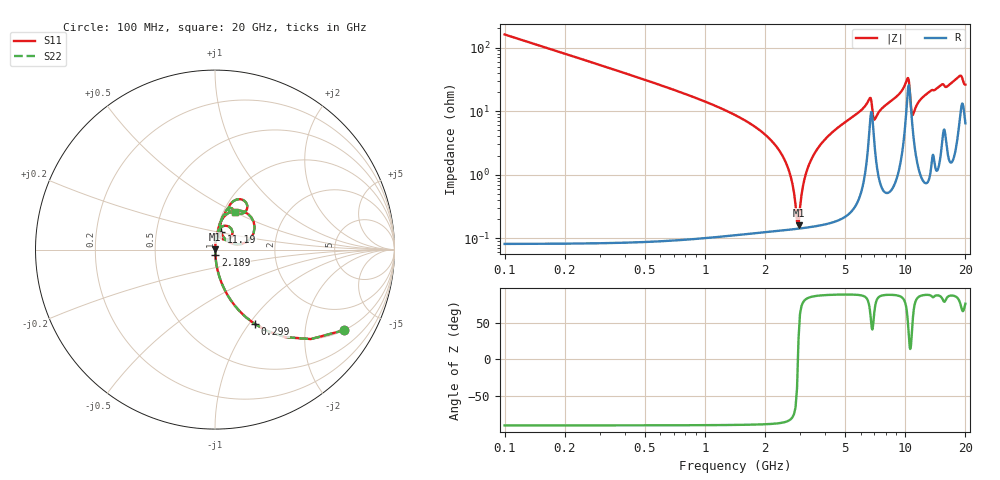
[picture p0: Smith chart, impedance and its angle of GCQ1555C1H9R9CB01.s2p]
!Murata Part Number: GCQ1555C1H9R9CB01
!These Parameters are Measured in Series Mode Connection
!Data Generated on Jan 08, 2026
!  o--ll--o
!Port1  Port2
!  o------o
!Operation Temp=25[degC], DC Bias Voltage=0[V]
!Freq. Start=100[MHz] Stop=20[GHz] 401[Steps]
# Hz S RI R 50
!Freq.(Hz) S11(Real) S11(Imag) S21(Real) S21(Imag) S12(Real) S12(Imag) S22(Real) S22(Imag)
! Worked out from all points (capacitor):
!   401 points, 100 MHz to 20 GHz, reference 50 ohm
!   read as one part in series: C = 9.9 pF near 199.5 MHz
!   lowest |Z| = 161 mohm at 2.936 GHz (marker M1)
!   series resonance near 2.916 GHz, so ESL is about 300 pH
!   S11 on the Smith chart (normalised r, x): 100 MHz: 1.00, -3.21; 299 MHz: 1.00, -1.06; 2.189 GHz: 1.00, -0.06; 11.19 GHz: 1.05, +0.21; 20 GHz: 1.13, +0.51
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1e8  0.7204 -0.4485  0.2796 0.4485  0.2796 0.4485  0.7204 -0.4485
2.99e8  0.221 -0.4141  0.779 0.4141  0.779 0.4141  0.221 -0.4141
7.4675e8  0.0397 -0.193  0.9603 0.193  0.9603 0.193  0.0397 -0.193
2.1895e9  0.00232 -0.0321  0.9977 0.0321  0.9977 0.0321  0.00232 -0.0321
2.5875e9  0.00153 -0.0133  0.9985 0.0133  0.9985 0.0133  0.00153 -0.0133
2.73675e9  0.00143 -0.00706  0.9986 0.00706  0.9986 0.00706  0.00143 -0.00706
2.83625e9  0.00141 -0.00309  0.9986 0.00309  0.9986 0.00309  0.00141 -0.00309
2.93575e9  0.00142 0.000746  0.9986 -0.000746  0.9986 -0.000746  0.00142 0.000746
3.1845e9  0.00156 0.00985  0.9984 -0.00985  0.9984 -0.00985  0.00156 0.00985
3.43325e9  0.00186 0.0184  0.9981 -0.0184  0.9981 -0.0184  0.00186 0.0184
4.478e9  0.00441 0.0506  0.9956 -0.0506  0.9956 -0.0506  0.00441 0.0506
6.61725e9  0.0618 0.133  0.9382 -0.133  0.9382 -0.133  0.0618 0.133
6.7665e9  0.0986 0.0956  0.9014 -0.0956  0.9014 -0.0956  0.0986 0.0956
7.065e9  0.0294 0.0667  0.9706 -0.0667  0.9706 -0.0667  0.0294 0.0667
1.005e10  0.1186 0.2179  0.8814 -0.2179  0.8814 -0.2179  0.1186 0.2179
1.039825e10  0.2207 0.1213  0.7793 -0.1213  0.7793 -0.1213  0.2207 0.1213
1.0846e10  0.0638 0.0522  0.9362 -0.0522  0.9362 -0.0522  0.0638 0.0522
1.119425e10  0.0348 0.0975  0.9652 -0.0975  0.9652 -0.0975  0.0348 0.0975
1.338325e10  0.0507 0.1949  0.9493 -0.1949  0.9493 -0.1949  0.0507 0.1949
1.67165e10  0.0781 0.2396  0.9219 -0.2396  0.9219 -0.2396  0.0781 0.2396
1.875625e10  0.16 0.2741  0.84 -0.2741  0.84 -0.2741  0.16 0.2741
2e10  0.1106 0.2111  0.8894 -0.2111  0.8894 -0.2111  0.1106 0.2111
